| IBIS file 100bga.ibs generated by Viper version: 2014.09.14
[IBIS Ver]   4.2
[Comment Char]   |_char
[File Name]   100bga.ibs
[File Rev]   1
[Date]   Mon Oct  5 12:20:01 2015
[Source]   FSL Viper 2014.09.14
[Notes]
   Single RLC values cover parasitic for all power pins
   (of a particular power domain) combined and hence
   if there are more than one power pin, RLC values are mentioned
   only for one pin and other power pins are commented
[Disclaimer] IMPORTANT NOTICE
  This information is provided on an AS IS basis and without warranty.
  IN NO EVENT SHALL Freescale BE LIABLE FOR INCIDENTAL OR CONSEQUENTIAL
  DAMAGES ARISING FROM USE OF THIS INFORMATION. THIS DISCLAIMER OF
  WARRANTY EXTENDS TO THE USER OF THE INFORMATION, AND TO THEIR CUSTOMERS
  OR USERS OF PRODUCTS  AND IS IN LIEU OF ALL WARRANTIES WHETHER EXPRESS,
  IMPLIED, OR STATUTORY, INCLUDING IMPLIED WARRANTIES OF MERCHANTABILITY
  OR FITNESS FOR PARTICULAR PURPOSE.
  Freescale does not represent or warrant that the information furnished
  hereunder is free of infringement of any third party patents,
  copyrights, trade secrets, or other intellectual property rights.
  Freescale does not represent or warrant that the information is free of
  defect, or that it meets any particular standard, requirements or need
  of the user of the infomation or their customers.
  Freescale reserves the right to change the information in this file
  without notice.
   http://www.freescale.com
[Copyright]   (C) Copyright Freescale 2004 - 2015, All Rights Reserved.
|   BGA100
[Component]   BGA100
[Manufacturer]   FREESCALE
[Package]
| variable   typ   min   max
R_pkg   0.1047590   0.0091279   0.315084
L_pkg   2.33705nH   0.25891nH   6.29081nH
C_pkg   0.97079pF   0.38181pF   5.45216pF
[Pin] signal_name   model_name   R_pin   L_pin   C_pin
A1   PI_0   pad_sr_hv   0.135114  2.60872nH 0.71670pF
A2   PI_1   pad_sr_hv   0.121415  2.3773nH  0.65722pF
A3   PI_3   pad_sr_hv   0.118039  2.38936nH 0.41182pF
A4   PORST   NC   0.108037  2.02152nH 0.61029pF
A5   PA_5   pad_sr_hv   0.0988514 2.14425nH 0.38181pF
A6   PE_15   pad_sr_hv   0.116521  2.35363nH 0.41890pF
A7   PG_14   pad_sr_hv   0.111892  2.37657nH 0.42196pF
A8   PF_15   pad_sr_hv   0.097714  3.05016nH 0.67724pF
A9   PE_13   pad_sr_hv   0.151696  3.35975nH 0.76157pF
A10   PA_7   pad_sr_hv   0.182577  3.64153nH 0.86424pF
B1   PG_2   pad_sr_hv   0.166051  3.46165nH 0.75570pF
B2   PG_3   pad_sr_hv   0.136851  2.83176nH 0.71411pF
B3   PI_2   pad_sr_hv   0.0732943 1.45063nH 0.43172pF
B4   PA_6   pad_sr_hv   0.0895012 2.34507nH 0.51139pF
B5   PH_12   pad_sr_hv   0.0875285 1.8454nH  0.45549pF
B6   PG_11   pad_sr_hv   0.0803852 1.67953nH 0.44346pF
B7   PG_15   pad_sr_hv   0.0732869 1.40366nH 0.39313pF
B8   PA_10   pad_sr_hv   0.129679  3.10038nH 0.49407pF
B9   PA_9   pad_sr_hv   0.106121  2.18072nH 0.49756pF
B10   PA_8   pad_sr_hv   0.0874746 1.80933nH 0.74565pF
C1   PE_9   pad_sr_hv   0.150456  3.26392nH 0.66962pF
C2   PE_8   pad_sr_hv   0.129905  3.31159nH 0.72224pF
C3   PE_2   pad_sr_hv   0.105472  2.3086nH  0.60071pF
C4   PH_9   pad_sr_hv   0.12473   2.55866nH 0.58510pF
C5   PC_0   pad_sr_hv   0.0919471 1.86306nH 0.53290pF
C6   PC_1   pad_sr_hv   0.0728814 1.43387nH 0.52977pF
C7   PH_10   pad_sr_hv   0.104307  2.5951nH  0.63665pF
C8   PA_11   pad_sr_hv   0.0863279 1.62837nH 0.56452pF
C9   PH_2   pad_sr_hv   0.0824464 2.188nH   0.57793pF
C10   PA_3   pad_sr_hv   0.134844  3.98166nH 0.69108pF
D1   VSS   GND   NA   NA   NA
D2   VPP   POWER   0.0822161 2.17171nH 0.51104pF
D3   PE_3   pad_sr_hv   0.151793  3.34216nH 0.65465pF
D4   VDD_HV_A   POWER   0.0091279 0.25891nH 5.45216pF
D5   VDD_LV   POWER   0.0147213 0.41158nH 3.90176pF
|D6   VDD_LV   POWER
|D7   VDD_HV_A   POWER
D8   PG_13   pad_sr_hv   0.101969  1.95866nH 0.53094pF
D9   PF_14   pad_sr_hv   0.0723425 1.3585nH  0.46619pF
D10   PG_12   pad_sr_hv   0.0921216 2.17246nH 0.52525pF
E1   VRC_CTRL   NC   0.142779  3.24189nH 0.42951pF
E2   INT_BAL_SELECT   NC   0.315084  6.29081nH 0.93981pF
E3   PC_5   pad_sr_hv   0.156586  3.64533nH 0.64332pF
E4   VSS   GND   NA   NA   NA
E5   VSS   GND   NA   NA   NA
E6   VSS   GND   NA   NA   NA
E7   VSS   GND   NA   NA   NA
E8   VDD_HV_B   POWER   0.0219772 0.57755nH 1.61656pF
E9   PH_1   pad_sr_hv   0.0695017 1.21471nH 0.48135pF
E10   PH_0   pad_sr_hv   0.0967859 2.10417nH 0.40271pF
F1   RESET   BD3MSCTFRESUDQ_5V0_65U_LIN   0.085353  1.49586nH 0.45049pF
F2   VDD_LP_DEC   POWER   0.102533  2.50287nH 0.51702pF
F3   PA_2   pad_sr_hv   0.124684  2.7596nH  0.89622pF
F4   VSS   GND   NA   NA   NA
F5   VSS   GND   NA   NA   NA
F6   VSS   GND   NA   NA   NA
F7   VSS   GND   NA   NA   NA
F8   PJ_0   pad_sr_hv   0.111529  2.9834nH  0.70388pF
F9   PG_0   pad_sr_hv   0.100521  2.59914nH 0.50693pF
F10   PG_1   pad_sr_hv   0.143437  3.85102nH 0.56504pF
G1   PC_11   pad_sr_hv   0.106942  2.32599nH 0.42129pF
G2   PC_10   pad_sr_hv   0.0818416 1.32139nH 0.44312pF
G3   PA_1   pad_sr_hv   0.150158  3.27709nH 0.74406pF
|G4   VDD_HV_A   POWER
|G5   VDD_LV   POWER
|G6   VDD_LV   POWER
|G7   VDD_HV_A   POWER
G8   PF_5   pad_sr_hv   0.167796  3.81342nH 0.68516pF
G9   PD_13   pad_sr_hv   0.0834465 1.29409nH 0.61766pF
G10   VDD_HV_ADC1   POWER   0.101384  2.21958nH 0.60245pF
H1   PB_1   pad_sr_hv   0.116575  2.64777nH 0.42886pF
H2   PB_0   pad_sr_hv   0.0844823 2.06396nH 0.43368pF
H3   VDD_HV_FLA   POWER   0.0931973 2.58327nH 0.64310pF
H4   PA_0   pad_sr_hv   0.189024  4.0506nH  0.70602pF
H5   PG_7   pad_sr_hv   0.162417  3.59644nH 0.76601pF
H6   PG_6   pad_sr_hv   0.192045  4.42421nH 0.77990pF
H7   PJ_2   pad_sr_hv   0.105218  2.13023nH 0.51879pF
H8   PJ_1   pad_sr_hv   0.110398  2.38734nH 0.59853pF
H9   VDD_HV_ADC1_REF   POWER   0.0832151 1.71464nH 0.47656pF
H10   VSS   GND   NA   NA   NA
J1   PF_9   pad_sr_hv   0.0914457 2.16384nH 0.62315pF
J2   PF_8   pad_sr_hv   0.100647  1.84314nH 0.73800pF
J3   PA_4   pad_sr_hv   0.0855599 1.63715nH 0.47469pF
J4   PA_15   pad_sr_hv   0.0771136 1.78614nH 0.52807pF
J5   PA_14   pad_sr_hv   0.0978684 2.99994nH 0.62214pF
J6   PA_13   pad_sr_hv   0.128507  2.94298nH 0.55512pF
J7   PA_12   pad_sr_hv   0.14353   3.65516nH 0.60651pF
J8   PF_0   pad_sr_hv   0.101706  2.89959nH 0.55651pF
J9   PI_14   pad_sr_hv   0.108567  2.09424nH 0.68685pF
J10   PD_1   ISATWINJUDQ_5V0_65U_LIN   0.135313  2.7819nH  0.60908pF
K1   PF_10   pad_sr_hv   0.137426  2.7559nH  0.74477pF
K2   PJ_14   pad_sr_hv   0.128311  3.0555nH  0.60655pF
K3   PJ_13   pad_sr_hv   0.103144  2.3303nH  0.48059pF
K4   VSS   GND   NA   NA   NA
K5   XTAL   NC   0.100713  1.9867nH  0.42678pF
K6   EXTAL   NC   0.104477  2.2721nH  0.42003pF
K7   VSS   GND   NA   NA   NA
K8   PB_10   pad_sr_hv   0.144651  3.27415nH 0.57070pF
K9   VSS   GND   NA   NA   NA
K10   VDD_HV_ADC0   POWER   0.0749606 2.47946nH 0.61287pF
[Pin Mapping]   pulldown_ref   pullup_ref
A1   VSS   VDD_HV_A
A2   VSS   VDD_HV_A
A3   VSS   VDD_HV_A
A4   NC   NC
A5   VSS   VDD_HV_A
A6   VSS   VDD_HV_A
A7   VSS   VDD_HV_A
A8   VSS   VDD_HV_B
A9   VSS   VDD_HV_B
A10   VSS   VDD_HV_B
B1   VSS   VDD_HV_A
B2   VSS   VDD_HV_A
B3   VSS   VDD_HV_A
B4   VSS   VDD_HV_A
B5   VSS   VDD_HV_A
B6   VSS   VDD_HV_A
B7   VSS   VDD_HV_A
B8   VSS   VDD_HV_B
B9   VSS   VDD_HV_B
B10   VSS   VDD_HV_B
C1   VSS   VDD_HV_A
C2   VSS   VDD_HV_A
C3   VSS   VDD_HV_A
C4   VSS   VDD_HV_A
C5   VSS   VDD_HV_A
C6   VSS   VDD_HV_A
C7   VSS   VDD_HV_A
C8   VSS   VDD_HV_B
C9   VSS   VDD_HV_B
C10   VSS   VDD_HV_B
D1   VSS   NC
D2   NC   VPP
D3   VSS   VDD_HV_A
D4   NC   VDD_HV_A
D5   NC   VDD_LV
D8   VSS   VDD_HV_B
D9   VSS   VDD_HV_B
D10   VSS   VDD_HV_B
E1   NC   NC
E2   NC   NC
E3   VSS   VDD_HV_A
E4   VSS   NC
E5   VSS   NC
E6   VSS   NC
E7   VSS   NC
E8   NC   VDD_HV_B
E9   VSS   VDD_HV_B
E10   VSS   VDD_HV_B
F1   VSS   VDD_HV_A
F2   NC   VDD_LP_DEC
F3   VSS   VDD_HV_A
F4   VSS   NC
F5   VSS   NC
F6   VSS   NC
F7   VSS   NC
F8   VSS   VDD_HV_A
F9   VSS   VDD_HV_B
F10   VSS   VDD_HV_B
G1   VSS   VDD_HV_A
G2   VSS   VDD_HV_A
G3   VSS   VDD_HV_A
G8   VSS   VDD_HV_A
G9   VSS   VDD_HV_A
G10   NC   VDD_HV_ADC1
H1   VSS   VDD_HV_A
H2   VSS   VDD_HV_A
H3   NC   VDD_HV_FLA
H4   VSS   VDD_HV_A
H5   VSS   VDD_HV_A
H6   VSS   VDD_HV_A
H7   VSS   VDD_HV_A
H8   VSS   VDD_HV_A
H9   NC   VDD_HV_ADC1_REF
H10   VSS   NC
J1   VSS   VDD_HV_A
J2   VSS   VDD_HV_A
J3   VSS   VDD_HV_A
J4   VSS   VDD_HV_A
J5   VSS   VDD_HV_A
J6   VSS   VDD_HV_A
J7   VSS   VDD_HV_A
J8   VSS   VDD_HV_A
J9   VSS   VDD_HV_A
J10   VSS   VDD_HV_A
K1   VSS   VDD_HV_A
K2   VSS   VDD_HV_A
K3   VSS   VDD_HV_A
K4   VSS   NC
K5   NC   NC
K6   NC   NC
K7   VSS   NC
K8   VSS   VDD_HV_A
K9   VSS   NC
K10   NC   VDD_HV_ADC0
|*   Model Selector   *
[Model Selector] BD3MSCTFRESUDQ_5V0_65U_LIN
BD3MSCTFRESUDQ_5V0_65U_LIN_0   ipp_ttl_lv=0 CMOS Receiver
BD3MSCTFRESUDQ_5V0_65U_LIN_1   ipp_ttl_lv=1 TTL  Receiver
[Model Selector] ISATWINJUDQ_5V0_65U_LIN
ISATWINJUDQ_5V0_65U_LIN_0   ipp_ttl_lv=0 ; Automotive mode receiver
ISATWINJUDQ_5V0_65U_LIN_1   ipp_ttl_lv=1 ; TTL receiver
[Model Selector] pad_sr_hv
sr11_5v   5V VDDE, full drive
sr11_3v   3.3V VDDE, full drive
sr10_5v   5V VDDE, half drive
sr10_3v   3.3V VDDE, half drive
srin_5v   5V VDDE, input
srin_3v   3.3V VDDE, input
| End [Component] BGA100
| Models and submodels in the file (10): BD3MSCTFRESUDQ_5V0_65U_LIN_0 (I/O_open_drain), BD3MSCTFRESUDQ_5V0_65U_LIN_1 (I/O_open_drain), ISATWINJUDQ_5V0_65U_LIN_0 (Input), ISATWINJUDQ_5V0_65U_LIN_1 (Input), sr10_3v (3-state), sr10_5v (3-state), sr11_3v (3-state), sr11_5v (3-state), srin_3v (Input), srin_5v (Input)
